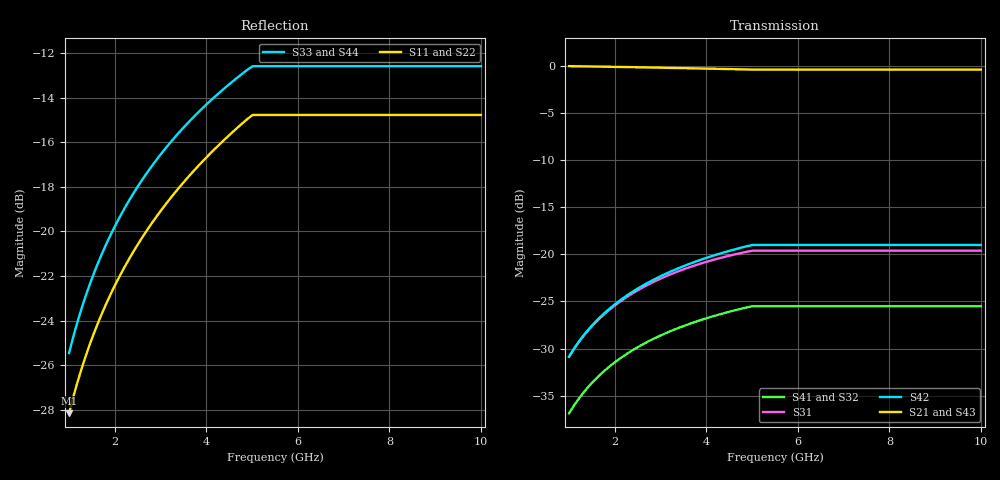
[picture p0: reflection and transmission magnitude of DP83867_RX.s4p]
! Created Fri May 12 13:45:50 2017
# hz S db R 50
! 4 Port Network Data from SP1.SP block
! freq  dbS11  angS11  dbS12  angS12  dbS13  angS13  dbS14  angS14
!  dbS21  angS21  dbS22  angS22  dbS23  angS23  dbS24  angS24
!  dbS31  angS31  dbS32  angS32  dbS33  angS33  dbS34  angS34
!  dbS41  angS41  dbS42  angS42  dbS43  angS43  dbS44  angS44
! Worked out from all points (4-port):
!   101 points, 1 GHz to 10 GHz, reference 50 ohm
!   strongest paths, dB at 1 GHz, 1.778 GHz, 3.162 GHz, 5.623 GHz, 10 GHz:
!     S21: -0.1, -0.1, -0.2, -0.4, -0.4
!     S43: -0.1, -0.1, -0.3, -0.6, -0.6
!     S42: -30.8, -26.2, -22.0, -19.0, -19.0
!     S31: -30.9, -26.3, -22.2, -19.6, -19.6
!     S41: -36.9, -32.3, -28.3, -25.5, -25.5
!     S32: -36.9, -32.3, -28.3, -25.6, -25.6
!   lowest |S11| = -28.2 dB at 1 GHz (marker M1), VSWR 1.08, Z = 51 + j3.81 ohm
!   |S11| at or under -10 dB: start of sweep to end of sweep
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1e9  -28.16 72.5  -0.06 -7.4  -30.88 76.0  -36.87 -110.2
     -0.06 -7.4  -28.22 81.7  -36.87 -110.4  -30.85 77.3
     -30.88 76.0  -36.87 -110.4  -25.46 73.5  -0.07 -8.0
     -36.87 -110.2  -30.85 77.3  -0.07 -8.0  -25.48 80.8
1.28825e9  -26.06 68.9  -0.08 -9.5  -28.83 72.8  -34.84 -115.1
           -0.08 -9.5  -26.14 80.9  -34.84 -115.3  -28.78 74.4
           -28.83 72.8  -34.84 -115.3  -23.36 69.9  -0.10 -10.2
           -34.84 -115.1  -28.78 74.4  -0.10 -10.2  -23.40 79.3
1.659587e9  -23.97 64.4  -0.10 -12.1  -26.85 68.7  -32.86 -121.3
            -0.10 -12.1  -24.07 79.8  -32.87 -121.5  -26.76 70.7
            -26.85 68.7  -32.87 -121.5  -21.28 65.3  -0.14 -13.0
            -32.86 -121.3  -26.76 70.7  -0.14 -13.0  -21.35 77.5
2.511886e9  -20.55 54.0  -0.17 -18.1  -23.79 60.1  -29.83 -134.7
            -0.17 -18.1  -20.74 77.5  -29.84 -135.0  -23.61 62.8
            -23.79 60.1  -29.84 -135.0  -17.95 55.1  -0.24 -19.4
            -29.83 -134.7  -23.61 62.8  -0.24 -19.4  -18.08 73.5
3.630781e9  -17.50 41.1  -0.28 -25.9  -21.38 50.0  -27.39 -150.8
            -0.28 -25.9  -17.78 75.0  -27.41 -151.1  -21.02 53.5
            -21.38 50.0  -27.41 -151.1  -15.06 42.3  -0.40 -27.5
            -27.39 -150.8  -21.02 53.5  -0.40 -27.5  -15.27 69.0
5.011872e9  -14.77 26.1  -0.42 -35.2  -19.62 39.2  -25.51 -169.0
            -0.42 -35.2  -15.14 72.2  -25.55 -169.4  -19.02 43.0
            -19.62 39.2  -25.55 -169.4  -12.59 27.7  -0.62 -37.1
            -25.51 -169.0  -19.02 43.0  -0.62 -37.1  -12.90 64.3
1e10  -14.77 26.1  -0.42 -35.2  -19.62 39.2  -25.51 -169.0
      -0.42 -35.2  -15.14 72.2  -25.55 -169.4  -19.02 43.0
      -19.62 39.2  -25.55 -169.4  -12.59 27.7  -0.62 -37.1
      -25.51 -169.0  -19.02 43.0  -0.62 -37.1  -12.90 64.3
